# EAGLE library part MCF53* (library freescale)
MCF537x ColdFire® Microprocessor Source: www.freescale.com .. MCF5373DS.pdf
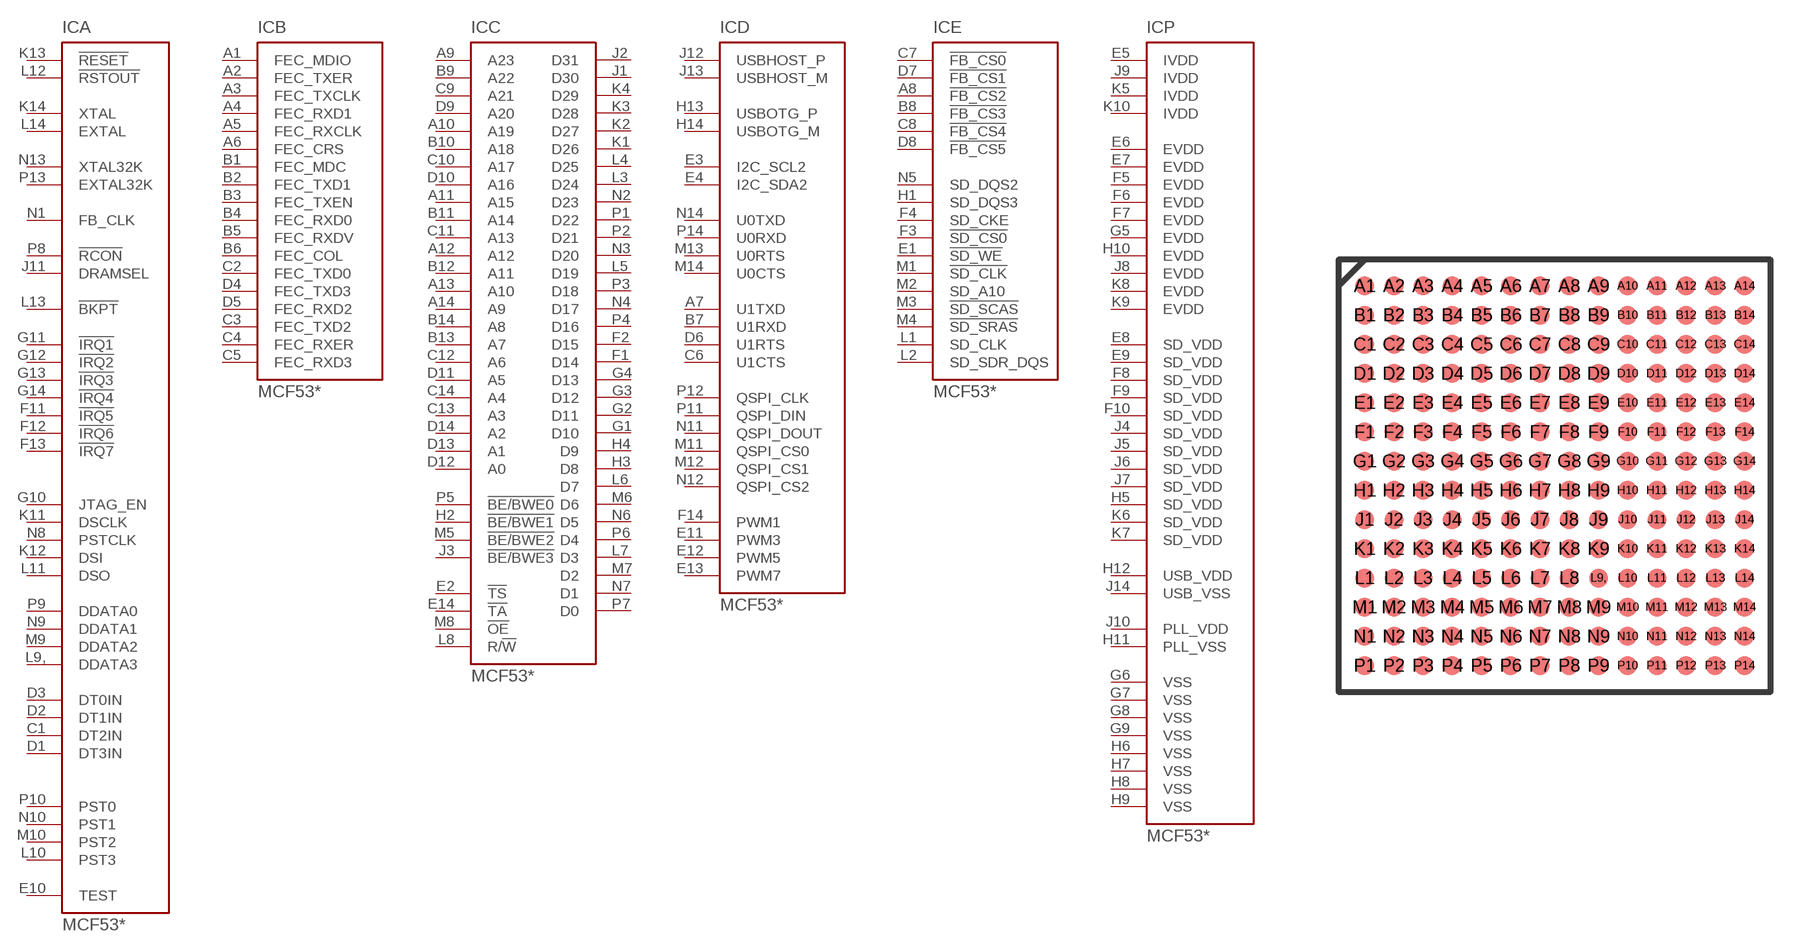
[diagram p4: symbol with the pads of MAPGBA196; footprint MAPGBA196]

Designator prefix IC; gates A=MCF537X-CONTROL B=MCF537X-FEC C=MCF537X-FLEXBUS D=MCF537X-IO E=MCF537X-SDRAM P=MCF537X-PWR

## MCF53271 (OC_FARNELL: unknown; OC_NEWARK: unknown), MCF5372L (MPN: MCF5372LCVM240J; OC_FARNELL: 1380411; OC_NEWARK: 57R6122), MCF5373L (MPN: MCF5373LCVM240J; OC_FARNELL: 1579871; OC_NEWARK: 57R6123)  [MAPGBA196]
A1  B:FEC_MDIO
A2  B:FEC_TXER  out
A3  B:FEC_TXCLK  in
A4  B:FEC_RXD1  in
A5  B:FEC_RXCLK  in
A6  B:FEC_CRS  in
A7  D:U1TXD  out
A8  E:!FB_CS2  out
A9  C:A23  out
A10  C:A19  out
A11  C:A15  out
A12  C:A12  out
A13  C:A10  out
A14  C:A9  out
B1  B:FEC_MDC  out
B2  B:FEC_TXD1  out
B3  B:FEC_TXEN  out
B4  B:FEC_RXD0  in
B5  B:FEC_RXDV  in
B6  B:FEC_COL  in
B7  D:U1RXD  in
B8  E:!FB_CS3  out
B9  C:A22  out
B10  C:A18  out
B11  C:A14  out
B12  C:A11  out
B13  C:A7  out
B14  C:A8  out
C1  A:DT2IN  in
C2  B:FEC_TXD0  out
C3  B:FEC_TXD2  out
C4  B:FEC_RXER  in
C5  B:FEC_RXD3  in
C6  D:U1CTS  in
C7  E:!FB_CS0  out
C8  E:!FB_CS4  out
C9  C:A21  out
C10  C:A17  out
C11  C:A13  out
C12  C:A6  out
C13  C:A3  out
C14  C:A4  out
D1  A:DT3IN  in
D2  A:DT1IN  in
D3  A:DT0IN  in
D4  B:FEC_TXD3  out
D5  B:FEC_RXD2  in
D6  D:U1RTS  out
D7  E:!FB_CS1  out
D8  E:!FB_CS5  out
D9  C:A20  out
D10  C:A16  out
D11  C:A5  out
D12  C:A0  out
D13  C:A1  out
D14  C:A2  out
E1  E:!SD_WE  out
E2  C:!TS  out
E3  D:I2C_SCL2
E4  D:I2C_SDA2
E5  P:IVDD  pwr
E6  P:EVDD  pwr
E7  P:EVDD  pwr
E8  P:SD_VDD  pwr
E9  P:SD_VDD  pwr
E10  A:TEST  in
E11  D:PWM3
E12  D:PWM5
E13  D:PWM7
E14  C:!TA  in
F1  C:D14
F2  C:D15
F3  E:!SD_CS0  out
F4  E:SD_CKE  out
F5  P:EVDD  pwr
F6  P:EVDD  pwr
F7  P:EVDD  pwr
F8  P:SD_VDD  pwr
F9  P:SD_VDD  pwr
F10  P:SD_VDD  pwr
F11  A:!IRQ5  in
F12  A:!IRQ6  in
F13  A:!IRQ7  in
F14  D:PWM1
G1  C:D10
G2  C:D11
G3  C:D12
G4  C:D13
G5  P:EVDD  pwr
G6  P:VSS  pwr
G7  P:VSS  pwr
G8  P:VSS  pwr
G9  P:VSS  pwr
G10  A:JTAG_EN  in
G11  A:!IRQ1  in
G12  A:!IRQ2  in
G13  A:!IRQ3  in
G14  A:!IRQ4  in
H1  E:SD_DQS3  out
H2  C:!BE/BWE1  out
H3  C:D8
H4  C:D9
H5  P:SD_VDD  pwr
H6  P:VSS  pwr
H7  P:VSS  pwr
H8  P:VSS  pwr
H9  P:VSS  pwr
H10  P:EVDD  pwr
H11  P:PLL_VSS  pwr
H12  P:USB_VDD  pwr
H13  D:USBOTG_P
H14  D:USBOTG_M
J1  C:D30
J2  C:D31
J3  C:!BE/BWE3  out
J4  P:SD_VDD  pwr
J5  P:SD_VDD  pwr
J6  P:SD_VDD  pwr
J7  P:SD_VDD  pwr
J8  P:EVDD  pwr
J9  P:IVDD  pwr
J10  P:PLL_VDD  pwr
J11  A:DRAMSEL  in
J12  D:USBHOST_P
J13  D:USBHOST_M
J14  P:USB_VSS  pwr
K1  C:D26
K2  C:D27
K3  C:D28
K4  C:D29
K5  P:IVDD  pwr
K6  P:SD_VDD  pwr
K7  P:SD_VDD  pwr
K8  P:EVDD  pwr
K9  P:EVDD  pwr
K10  P:IVDD  pwr
K11  A:DSCLK  in
K12  A:DSI  in
K13  A:!RESET  in
K14  A:XTAL  out
L1  E:SD_CLK  out
L2  E:SD_SDR_DQS  out
L3  C:D24
L4  C:D25
L5  C:D19
L6  C:D7
L7  C:D3
L8  C:R/!W  out
L9,  A:DDATA3  out
L10  A:PST3  out
L11  A:DSO  out
L12  A:!RSTOUT  out
L13  A:!BKPT  in
L14  A:EXTAL  in
M1  E:!SD_CLK  out
M2  E:SD_A10  out
M3  E:!SD_SCAS  out
M4  E:!SD_SRAS  out
M5  C:!BE/BWE2  out
M6  C:D6
M7  C:D2
M8  C:!OE  out
M9  A:DDATA2  out
M10  A:PST2  out
M11  D:QSPI_CS0  out
M12  D:QSPI_CS1  out
M13  D:U0RTS  out
M14  D:U0CTS  in
N1  A:FB_CLK  out
N2  C:D23
N3  C:D20
N4  C:D17
N5  E:SD_DQS2  out
N6  C:D5
N7  C:D1
N8  A:PSTCLK  out
N9  A:DDATA1  out
N10  A:PST1  out
N11  D:QSPI_DOUT  out
N12  D:QSPI_CS2  out
N13  A:XTAL32K  out
N14  D:U0TXD  out
P1  C:D22
P2  C:D21
P3  C:D18
P4  C:D16
P5  C:!BE/BWE0  out
P6  C:D4
P7  C:D0
P8  A:!RCON  in
P9  A:DDATA0  out
P10  A:PST0  out
P11  D:QSPI_DIN  in
P12  D:QSPI_CLK  out
P13  A:EXTAL32K  in
P14  D:U0RXD  in

## Footprint MAPGBA196 (pad centres in mm)
smd 0.65 x 0.65: A1 -6.5,6.5; A2 -5.5,6.5; A3 -4.5,6.5; A4 -3.5,6.5; A5 -2.5,6.5; A6 -1.5,6.5; A7 -0.5,6.5; A8 0.5,6.5; A9 1.5,6.5; A10 2.5,6.5; A11 3.5,6.5; A12 4.5,6.5; A13 5.5,6.5; A14 6.5,6.5; B1 -6.5,5.5; B2 -5.5,5.5; B3 -4.5,5.5; B4 -3.5,5.5; B5 -2.5,5.5; B6 -1.5,5.5; B7 -0.5,5.5; B8 0.5,5.5; B9 1.5,5.5; B10 2.5,5.5; B11 3.5,5.5; B12 4.5,5.5; B13 5.5,5.5; B14 6.5,5.5; C1 -6.5,4.5; C2 -5.5,4.5; C3 -4.5,4.5; C4 -3.5,4.5; C5 -2.5,4.5; C6 -1.5,4.5; C7 -0.5,4.5; C8 0.5,4.5; C9 1.5,4.5; C10 2.5,4.5; C11 3.5,4.5; C12 4.5,4.5; C13 5.5,4.5; C14 6.5,4.5; D1 -6.5,3.5; D2 -5.5,3.5; D3 -4.5,3.5; D4 -3.5,3.5; D5 -2.5,3.5; D6 -1.5,3.5; D7 -0.5,3.5; D8 0.5,3.5; D9 1.5,3.5; D10 2.5,3.5; D11 3.5,3.5; D12 4.5,3.5; D13 5.5,3.5; D14 6.5,3.5; E1 -6.5,2.5; E2 -5.5,2.5; E3 -4.5,2.5; E4 -3.5,2.5; E5 -2.5,2.5; E6 -1.5,2.5; E7 -0.5,2.5; E8 0.5,2.5; E9 1.5,2.5; E10 2.5,2.5; E11 3.5,2.5; E12 4.5,2.5; E13 5.5,2.5; E14 6.5,2.5; F1 -6.5,1.5; F2 -5.5,1.5; F3 -4.5,1.5; F4 -3.5,1.5; F5 -2.5,1.5; F6 -1.5,1.5; F7 -0.5,1.5; F8 0.5,1.5; F9 1.5,1.5; F10 2.5,1.5; F11 3.5,1.5; F12 4.5,1.5; F13 5.5,1.5; F14 6.5,1.5; G1 -6.5,0.5; G2 -5.5,0.5; G3 -4.5,0.5; G4 -3.5,0.5; G5 -2.5,0.5; G6 -1.5,0.5; G7 -0.5,0.5; G8 0.5,0.5; G9 1.5,0.5; G10 2.5,0.5; G11 3.5,0.5; G12 4.5,0.5; G13 5.5,0.5; G14 6.5,0.5; H1 -6.5,-0.5; H2 -5.5,-0.5; H3 -4.5,-0.5; H4 -3.5,-0.5; H5 -2.5,-0.5; H6 -1.5,-0.5; H7 -0.5,-0.5; H8 0.5,-0.5; H9 1.5,-0.5; H10 2.5,-0.5; H11 3.5,-0.5; H12 4.5,-0.5; H13 5.5,-0.5; H14 6.5,-0.5; J1 -6.5,-1.5; J2 -5.5,-1.5; J3 -4.5,-1.5; J4 -3.5,-1.5; J5 -2.5,-1.5; J6 -1.5,-1.5; J7 -0.5,-1.5; J8 0.5,-1.5; J9 1.5,-1.5; J10 2.5,-1.5; J11 3.5,-1.5; J12 4.5,-1.5; J13 5.5,-1.5; J14 6.5,-1.5; K1 -6.5,-2.5; K2 -5.5,-2.5; K3 -4.5,-2.5; K4 -3.5,-2.5; K5 -2.5,-2.5; K6 -1.5,-2.5; K7 -0.5,-2.5; K8 0.5,-2.5; K9 1.5,-2.5; K10 2.5,-2.5; K11 3.5,-2.5; K12 4.5,-2.5; K13 5.5,-2.5; K14 6.5,-2.5; L1 -6.5,-3.5; L2 -5.5,-3.5; L3 -4.5,-3.5; L4 -3.5,-3.5; L5 -2.5,-3.5; L6 -1.5,-3.5; L7 -0.5,-3.5; L8 0.5,-3.5; L9, 1.5,-3.5; L10 2.5,-3.5; L11 3.5,-3.5; L12 4.5,-3.5; L13 5.5,-3.5; L14 6.5,-3.5; M1 -6.5,-4.5; M2 -5.5,-4.5; M3 -4.5,-4.5; M4 -3.5,-4.5; M5 -2.5,-4.5; M6 -1.5,-4.5; M7 -0.5,-4.5; M8 0.5,-4.5; M9 1.5,-4.5; M10 2.5,-4.5; M11 3.5,-4.5; M12 4.5,-4.5; M13 5.5,-4.5; M14 6.5,-4.5; N1 -6.5,-5.5; N2 -5.5,-5.5; N3 -4.5,-5.5; N4 -3.5,-5.5; N5 -2.5,-5.5; N6 -1.5,-5.5; N7 -0.5,-5.5; N8 0.5,-5.5; N9 1.5,-5.5; N10 2.5,-5.5; N11 3.5,-5.5; N12 4.5,-5.5; N13 5.5,-5.5; N14 6.5,-5.5; P1 -6.5,-6.5; P2 -5.5,-6.5; P3 -4.5,-6.5; P4 -3.5,-6.5; P5 -2.5,-6.5; P6 -1.5,-6.5; P7 -0.5,-6.5; P8 0.5,-6.5; P9 1.5,-6.5; P10 2.5,-6.5; P11 3.5,-6.5; P12 4.5,-6.5; P13 5.5,-6.5; P14 6.5,-6.5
